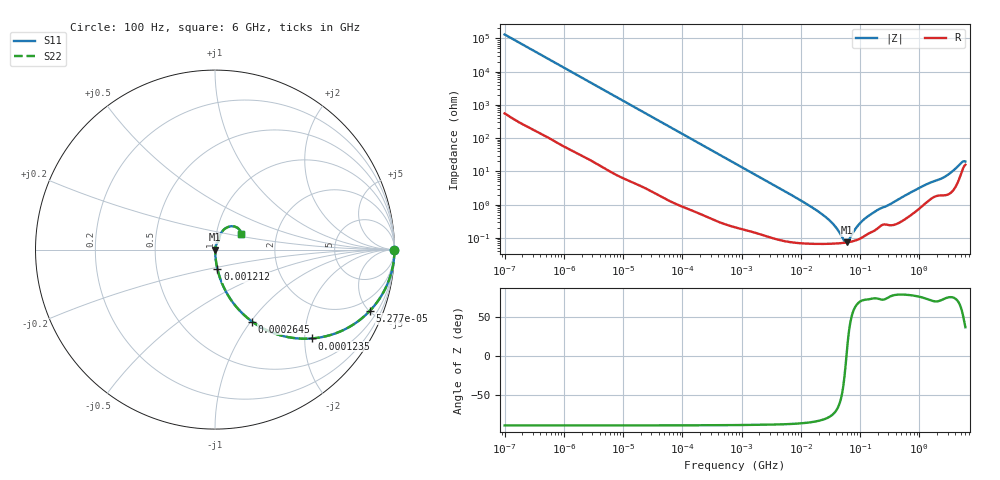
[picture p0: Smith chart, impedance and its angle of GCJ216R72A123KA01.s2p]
!Murata Part Number: GCJ216R72A123KA01
!These Parameters are Measured in Series Mode Connection
!Data Generated on Mar 13, 2026
!  o--ll--o
!Port1  Port2
!  o------o
!Operation Temp=25[degC], DC Bias Voltage=0[V]
!Freq. Start=100[Hz] Stop=6[GHz] 401[Steps]
# Hz S RI R 50
!Freq.(Hz) S11(Real) S11(Imag) S21(Real) S21(Imag) S12(Real) S12(Imag) S22(Real) S22(Imag)
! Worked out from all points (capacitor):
!   401 points, 100 Hz to 6 GHz, reference 50 ohm
!   read as one part in series: C = 12.1 nF near 109 Hz
!   lowest |Z| = 72.9 mohm at 59.6 MHz (marker M1)
!   series resonance near 58.93 MHz, so ESL is about 600 pH
!   S11 on the Smith chart (normalised r, x): 100 Hz: open; 52.77 kHz: 1.03, -5.06; 123.5 kHz: 1.01, -2.17; 264.5 kHz: 1.01, -1.02; 1.212 MHz: 1.00, -0.22; 6 GHz: 1.32, +0.24
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100  1 -0.000763  3.8e-06 0.000763  3.8e-06 0.000763  1 -0.000763
2008  0.9997 -0.0152  0.0003 0.0152  0.0003 0.0152  0.9997 -0.0152
12041  0.9914 -0.0899  0.00859 0.0899  0.00859 0.0899  0.9914 -0.0899
40335  0.9148 -0.2763  0.0852 0.2763  0.0852 0.2763  0.9148 -0.2763
52766  0.8633 -0.3406  0.1367 0.3406  0.1367 0.3406  0.8633 -0.3406
123542  0.5395 -0.495  0.4605 0.495  0.4605 0.495  0.5395 -0.495
264476  0.2069 -0.4009  0.7931 0.4009  0.7931 0.4009  0.2069 -0.4009
774597  0.0313 -0.1683  0.9687 0.1683  0.9687 0.1683  0.0313 -0.1683
1212075  0.0139 -0.1098  0.9861 0.1098  0.9861 0.1098  0.0139 -0.1098
1.555665e7  0.000728 -0.00819  0.9993 0.00819  0.9993 0.00819  0.000728 -0.00819
3.184506e7  0.000673 -0.00305  0.9993 0.00305  0.9993 0.00305  0.000673 -0.00305
3.983537e7  0.00068 -0.00187  0.9993 0.00187  0.9993 0.00187  0.00068 -0.00187
5.449875e7  0.000711 -0.000364  0.9993 0.000364  0.9993 0.000364  0.000711 -0.000364
5.960426e7  0.000726 5.4e-05  0.9993 -5.4e-05  0.9993 -5.4e-05  0.000726 5.4e-05
8.918374e7  0.000871 0.002  0.9991 -0.002  0.9991 -0.002  0.000871 0.002
1.166697e8  0.00112 0.00343  0.9989 -0.00343  0.9989 -0.00343  0.00112 0.00343
1.996653e8  0.002 0.00669  0.998 -0.00669  0.998 -0.00669  0.002 0.00669
3.124326e8  0.00249 0.00964  0.9975 -0.00964  0.9975 -0.00964  0.00249 0.00964
9.569533e8  0.00791 0.0293  0.9921 -0.0293  0.9921 -0.0293  0.00791 0.0293
3.352442e9  0.0288 0.0827  0.9712 -0.0827  0.9712 -0.0827  0.0288 0.0827
5.016141e9  0.0924 0.1302  0.9076 -0.1302  0.9076 -0.1302  0.0924 0.1302
6e9  0.1455 0.0875  0.8545 -0.0875  0.8545 -0.0875  0.1455 0.0875
